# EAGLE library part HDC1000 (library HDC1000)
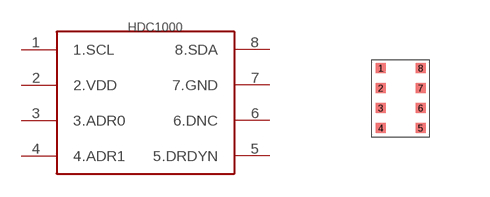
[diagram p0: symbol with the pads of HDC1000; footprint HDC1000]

Designator prefix -

## HDC1000  [HDC1000]
1  1.SCL
2  2.VDD
3  3.ADR0
4  4.ADR1
5  5.DRDYN
6  6.DNC
7  7.GND
8  8.SDA

## Footprint HDC1000 (pad centres in mm)
smd 0.25 x 0.25: 1 0,0; 2 0,-0.5; 3 0,-1; 4 0,-1.5; 5 1,-1.5; 6 1,-1; 7 1,-0.5; 8 1,0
